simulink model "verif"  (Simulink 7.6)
settings: Solver=ode15s  StartTime=0.0  StopTime=0.02  RelTol=1e-3
InitFcn:
  | N=2000;
libraries: fl_lib x11, nesl_utility x6, dspstat3 x2

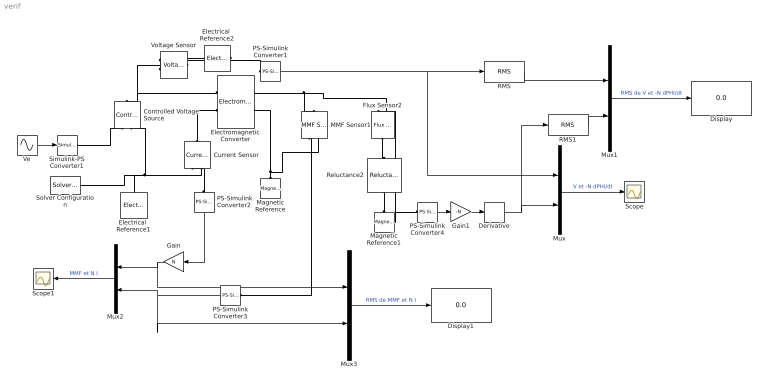
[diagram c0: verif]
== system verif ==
  Controlled Voltage Source : fl_lib/Electrical/Electrical Sources/Controlled Voltage Source  DialogController=NetworkEngine.DynNeDlgSource  SystemSampleTime=-1  i_Log=off  v_Log=off  LocalVarNames=|i|v  LocalVarDescs=|i|v  LocalVarLogging=[0 0]
  Current Sensor : fl_lib/Electrical/Electrical Sensors/Current Sensor  DialogController=NetworkEngine.DynNeDlgSource  SystemSampleTime=-1  i1_Log=off  v1_Log=off  LocalVarNames=|i1|v1  LocalVarDescs=|i1|v1  LocalVarLogging=[0 0]
  Derivative : Derivative
  Display : Display
  Display1 : Display
  Electrical  Reference1 : fl_lib/Electrical/Electrical Elements/Electrical Reference  DialogController=NetworkEngine.DynNeDlgSource  SystemSampleTime=-1  i_Log=off  LocalVarNames=|i  LocalVarDescs=|i  LocalVarLogging=0
  Electrical  Reference2 : fl_lib/Electrical/Electrical Elements/Electrical Reference  DialogController=NetworkEngine.DynNeDlgSource  SystemSampleTime=-1  i_Log=off  LocalVarNames=|i  LocalVarDescs=|i  LocalVarLogging=0
  Electromagnetic Converter : fl_lib/Magnetic/Magnetic Elements/Electromagnetic Converter  DialogController=NetworkEngine.DynNeDlgSource  SystemSampleTime=-1  Nw=N  i_Log=off  v_Log=off  mmf_Log=off  phi_Log=off  LocalVarNames=|i|v|mmf|phi  LocalVarDescs=|i|v|mmf|phi  LocalVarLogging=[0 0 0 0]
  Flux Sensor2 : fl_lib/Magnetic/Magnetic Sensors/Flux Sensor  DialogController=NetworkEngine.DynNeDlgSource  SystemSampleTime=-1  phi_Log=off  mmf_Log=off  LocalVarNames=|phi|mmf  LocalVarDescs=|phi|mmf  LocalVarLogging=[0 0]
  Gain : Gain  Gain=N
  Gain1 : Gain  Gain=-N
  MMF Sensor1 : fl_lib/Magnetic/Magnetic Sensors/MMF Sensor  DialogController=NetworkEngine.DynNeDlgSource  SystemSampleTime=-1  phi_Log=off  mmf_Log=off  LocalVarNames=|phi|mmf  LocalVarDescs=|phi|mmf  LocalVarLogging=[0 0]
  Magnetic Reference : fl_lib/Magnetic/Magnetic Elements/Magnetic Reference  DialogController=NetworkEngine.DynNeDlgSource  SystemSampleTime=-1  phi_Log=off  LocalVarNames=|phi  LocalVarDescs=|phi  LocalVarLogging=0
  Magnetic Reference1 : fl_lib/Magnetic/Magnetic Elements/Magnetic Reference  DialogController=NetworkEngine.DynNeDlgSource  SystemSampleTime=-1  phi_Log=off  LocalVarNames=|phi  LocalVarDescs=|phi  LocalVarLogging=0
  Mux{,1..3} (4 alike) : Mux  Inputs=2
  PS-Simulink Converter1 : nesl_utility/PS-Simulink Converter  DialogController=NetworkEngine.DynNeUtilDlgSource  SystemSampleTime=-1  PhysicalDomain=network_engine_domain  LeftPortType=input  RightPortType=output  SubClassName=ps_output  Unit=V  AffineConversion=off
  PS-Simulink Converter2 : nesl_utility/PS-Simulink Converter  DialogController=NetworkEngine.DynNeUtilDlgSource  SystemSampleTime=-1  PhysicalDomain=network_engine_domain  LeftPortType=input  RightPortType=output  SubClassName=ps_output  Unit=1  AffineConversion=off
  PS-Simulink Converter3 : nesl_utility/PS-Simulink Converter  DialogController=NetworkEngine.DynNeUtilDlgSource  SystemSampleTime=-1  PhysicalDomain=network_engine_domain  LeftPortType=input  RightPortType=output  SubClassName=ps_output  Unit=1  AffineConversion=off
  PS-Simulink Converter4 : nesl_utility/PS-Simulink Converter  DialogController=NetworkEngine.DynNeUtilDlgSource  SystemSampleTime=-1  PhysicalDomain=network_engine_domain  LeftPortType=input  RightPortType=output  SubClassName=ps_output  Unit=Wb  AffineConversion=off
  RMS : dspstat3/RMS  DialogController=dspDDGCreate  DialogControllerArgs=DataTag1  run=off  reset_popup=None  InputProcessing=Columns as channels (frame based)  directionMode=Each column  dimension=1  treatSBRowAsCol=on
  RMS1 : dspstat3/RMS  DialogController=dspDDGCreate  DialogControllerArgs=DataTag3  run=off  reset_popup=None  InputProcessing=Columns as channels (frame based)  directionMode=Each column  dimension=1  treatSBRowAsCol=on
  Reluctance2 : fl_lib/Magnetic/Magnetic Elements/Reluctance  DialogController=NetworkEngine.DynNeDlgSource  SystemSampleTime=-1  g=0.001 m  CSA=0.01 m^2  mur=1  phi_Log=off  mmf_Log=off  LocalVarNames=|phi|mmf  LocalVarDescs=|phi|mmf  LocalVarLogging=[0 0]
  Scope : Scope
  Scope1 : Scope
  Simulink-PS Converter1 : nesl_utility/Simulink-PS Converter  DialogController=NetworkEngine.DynNeUtilDlgSource  SystemSampleTime=-1  PhysicalDomain=network_engine_domain  LeftPortType=input  RightPortType=output  SubClassName=ps_input  Unit=1  AffineConversion=off  InputFilterTimeConstant=.001  UdotUserProvided=0
  Solver Configuration : nesl_utility/Solver Configuration  DialogController=NetworkEngine.DynNeUtilDlgSource  SystemSampleTime=-1  PhysicalDomain=network_engine_domain  LeftPortType=input  RightPortType=generic  SubClassName=solver  Accelerate=off  Profile=off  ResidualTolerance=1e-9  MaxNonlinIter=3  MaxModeIter=2  DoFixedCost=off  UseLocalSampling=off  DoDC=off  LinearAlgebra=Sparse  LocalSolverSampleTime=.001  LocalSolverChoice=NE_BACKWARD_EULER_ADVANCER  UseLocalSolver=off
  Ve : Sin  Amplitude=120  Frequency=4*pi*60  Phase=pi/2  SampleTime=0
  Voltage Sensor : fl_lib/Electrical/Electrical Sensors/Voltage Sensor  DialogController=NetworkEngine.DynNeDlgSource  SystemSampleTime=-1  i1_Log=off  v1_Log=off  LocalVarNames=|i1|v1  LocalVarDescs=|i1|v1  LocalVarLogging=[0 0]
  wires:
  Ve/1 -> Simulink-PS Converter1/1
  Mux/1 -> Scope/1  "V et -N dPHI/dt"
  PS-Simulink Converter2/1 -> Gain/1
  Gain/1 -> Mux2/1, Mux3/1
  PS-Simulink Converter3/1 -> Mux2/2, Mux3/2
  PS-Simulink Converter4/1 -> Gain1/1
  PS-Simulink Converter1/1 -> Mux/1, RMS/1
  Gain1/1 -> Derivative/1
  Derivative/1 -> Mux/2, RMS1/1
  Mux2/1 -> Scope1/1  "MMF et N I"
  RMS/1 -> Mux1/1
  RMS1/1 -> Mux1/2
  Mux1/1 -> Display/1  "RMS de V et -N dPHI/dt"
  Mux3/1 -> Display1/1  "RMS de MMF et N I"
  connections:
  Electromagnetic Converter/RConn1 -- MMF Sensor1/LConn1 -- Flux Sensor2/RConn2
  Magnetic Reference/LConn1 -- Electromagnetic Converter/RConn2 -- MMF Sensor1/RConn2
  Simulink-PS Converter1/RConn1 -- Controlled Voltage Source/RConn1
  Electromagnetic Converter/LConn1 -- Controlled Voltage Source/LConn1 -- Voltage Sensor/LConn1
  Current Sensor/RConn2 -- Electrical  Reference1/LConn1 -- Controlled Voltage Source/RConn2 -- Solver Configuration/RConn1
  Current Sensor/LConn1 -- Electromagnetic Converter/LConn2
  PS-Simulink Converter1/LConn1 -- Voltage Sensor/RConn1
  PS-Simulink Converter2/LConn1 -- Current Sensor/RConn1
  PS-Simulink Converter3/LConn1 -- MMF Sensor1/RConn1
  Voltage Sensor/RConn2 -- Electrical  Reference2/LConn1
  Reluctance2/LConn1 -- Magnetic Reference1/LConn1
  Flux Sensor2/LConn1 -- Reluctance2/RConn1
  Flux Sensor2/RConn1 -- PS-Simulink Converter4/LConn1
